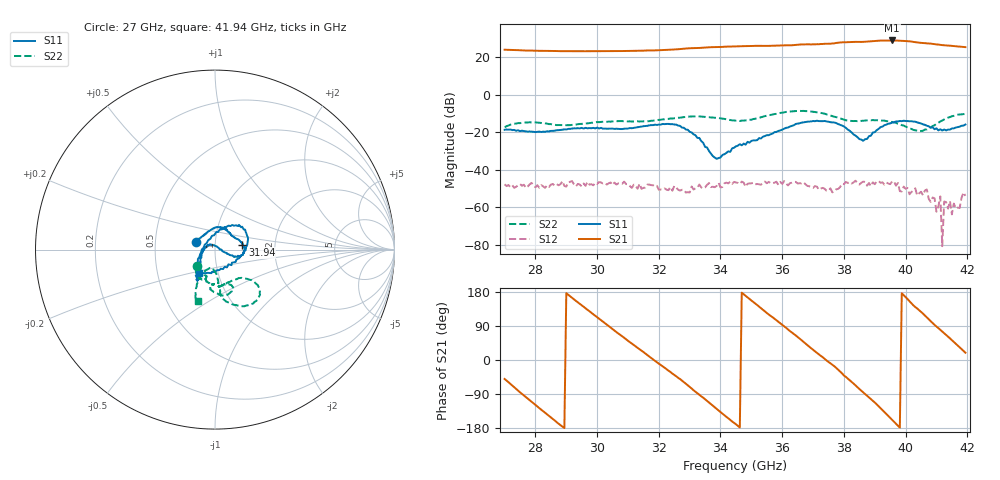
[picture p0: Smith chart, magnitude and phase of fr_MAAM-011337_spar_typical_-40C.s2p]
! Created Thu Jan 25 15:57:36 2024
# hz S db R 50
! 2 Port Network Data from SP1.SP block
! freq  dbS11  angS11  dbS21  angS21  dbS12  angS12  dbS22  angS22
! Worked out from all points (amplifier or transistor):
!   240 points, 27 GHz to 41.94 GHz, reference 50 ohm
!   highest |S21| = 28.8 dB at 39.56 GHz (marker M1)
!   |S21| within 3 dB of that: 34.84 GHz to 41.56 GHz (6.726 GHz wide, 17.6 % of centre)
!   unconditionally stable (mu >= 1): start of sweep to end of sweep
!   at 29.5 GHz: K = 9.41, MAG = 23.3 dB, |S12| = -48.9 dB
!   at 34.5 GHz: K = 5.55, MAG = 25.8 dB, |S12| = -46.9 dB
!   at 41.94 GHz: K = 12.09, MAG = 25.8 dB, |S12| = -53.9 dB
!   S11 on the Smith chart (normalised r, x): 27 GHz: 0.80, +0.07; 31.94 GHz: 1.36, +0.08; 41.94 GHz: 0.81, -0.22
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2.70046e10  -18.76 159.0  23.88 -50.0  -47.81 -102.5  -17.39 -136.9
2.762948e10  -19.46 144.2  23.50 -93.6  -48.03 -132.7  -14.97 -119.9
2.844181e10  -19.63 113.8  23.24 -147.4  -49.20 -157.3  -15.74 -107.0
2.95041e10  -17.76 76.5  23.06 144.5  -48.94 169.3  -15.62 -110.7
3.062888e10  -18.19 45.6  23.16 73.6  -47.94 130.0  -14.21 -94.8
3.194111e10  -16.21 10.1  23.56 -5.9  -48.64 76.0  -13.66 -97.3
3.20036e10  -15.99 9.6  23.61 -9.7  -50.68 88.6  -13.48 -97.2
3.344081e10  -25.72 -14.6  25.03 -99.5  -50.02 64.2  -11.83 -71.7
3.45031e10  -27.60 136.5  25.66 -169.6  -46.86 25.4  -13.92 -72.1
3.512798e10  -24.45 -179.1  25.94 148.8  -47.83 24.5  -12.89 -82.9
3.587782e10  -19.37 -138.1  26.11 101.0  -48.14 -3.8  -9.97 -72.9
3.65027e10  -15.46 -120.3  26.52 60.6  -47.35 -26.9  -8.76 -56.4
3.70026e10  -14.10 -120.2  26.78 27.1  -49.67 -44.3  -9.16 -44.4
3.781494e10  -15.66 -130.0  27.62 -25.6  -50.29 -34.9  -12.34 -42.3
3.843981e10  -22.70 179.3  28.03 -71.9  -47.13 -76.7  -14.17 -68.5
3.90022e10  -20.04 80.0  28.60 -112.1  -47.75 -95.8  -13.71 -83.4
3.95021e10  -15.37 51.4  28.81 -153.0  -47.72 -121.1  -14.58 -84.0
3.956459e10  -14.96 49.4  28.81 -157.8  -46.27 -121.8  -14.58 -84.9
4.006449e10  -14.12 27.4  28.41 160.9  -49.77 -157.4  -17.47 -86.9
4.075185e10  -16.91 -19.5  27.22 107.9  -55.56 141.7  -17.81 -114.8
4.131424e10  -19.09 -73.4  26.19 66.4  -57.29 33.3  -12.79 -116.3
4.193911e10  -15.96 -125.1  25.26 19.3  -53.93 -65.8  -10.41 -108.5
